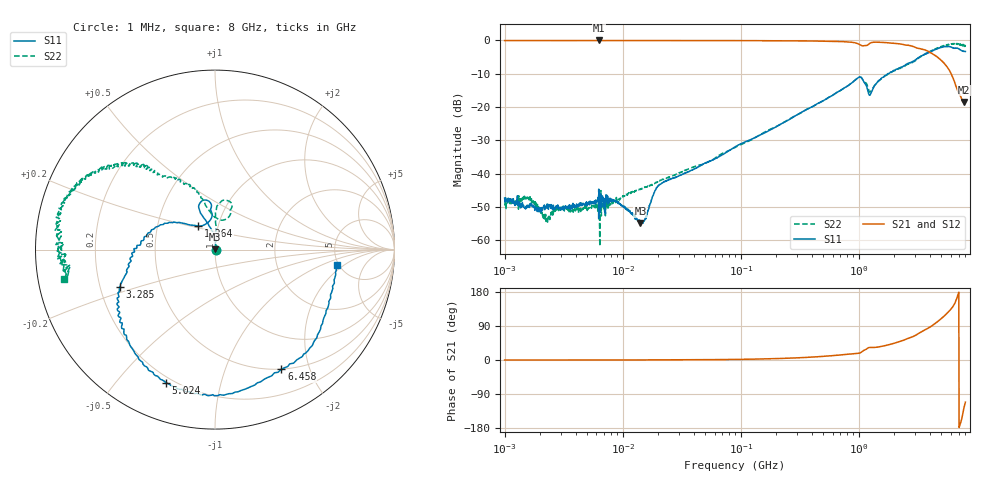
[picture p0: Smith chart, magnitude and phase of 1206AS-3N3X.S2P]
!s-Parameter Generated by FASTRON Sdn. Bhd.
!FASTRON P/N : 1206AS-3N3X
!Keysight Technologies: E5071C_MY46733604_B.14.02
!Date: Wed Nov 15 09:28:28 2023
!Version  :Rev00  Wed Nov 15 09:28:28 2023
!Data & Calibration Information:
!Freq  S11:SOLT2(ON)  S21:SOLT2(ON)  S12:SOLT2(ON)  S22:SOLT2(ON)
!PortZ  Port1:50+j0  Port2:50+j0
!When reading reference impedance value at option line is always used.
! Remarks : This data is being provided solely for informational purposes.
# Hz S dB R 50
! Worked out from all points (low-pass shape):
!   1601 points, 1 MHz to 8 GHz, reference 50 ohm
!   highest |S21| = 0.00 dB at 6.301 MHz (marker M1); lowest = -18.5 dB at 7.769 GHz (marker M2)
!   |S21| within 3 dB of the highest: start of sweep to 3.704 GHz
!   lowest |S11| = -54.9 dB at 14.15 MHz (marker M3), VSWR 1.00, Z = 50.1 + j0.125 ohm
!   |S11| at or under -10 dB: start of sweep to 1.756 GHz
!   |S22| runs from -61.8 to -0.9 dB; largest |S21 - S12| = 0.0043
!   S11 on the Smith chart (normalised r, x): 1 MHz: 1.01, -0.00; 1.264 GHz: 0.81, +0.22; 3.285 GHz: 0.28, -0.18; 5.024 GHz: 0.17, -0.68; 6.458 GHz: 0.50, -1.59; 8 GHz: 4.79, -1.55
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1000000  -47.36 -27.2  -0.02 -0.1  -0.04 -0.1  -49.23 -33.5
1568286  -50.06 -31.4  -0.02 -0.1  -0.03 -0.0  -47.04 -37.2
2286470  -49.17 8.8  -0.03 -0.0  -0.03 -0.0  -53.57 13.9
2905262  -50.51 4.0  -0.03 -0.0  -0.03 0.0  -50.89 1.5
4479405  -48.96 16.8  -0.03 0.0  -0.04 0.0  -50.94 21.6
6301378  -44.76 8.2  0.00 -0.1  -0.02 0.1  -49.76 -41.4
8860562  -48.44 31.0  -0.03 0.1  -0.03 0.1  -47.19 33.3
1.414737e7  -54.90 44.0  -0.03 0.2  -0.04 0.2  -44.58 35.3
1.552719e7  -53.42 55.5  -0.03 0.2  -0.04 0.2  -44.08 38.7
2.00676e7  -43.55 56.6  -0.03 0.3  -0.04 0.4  -42.34 57.9
8.994653e7  -31.93 81.2  -0.05 1.5  -0.06 1.5  -32.14 77.8
4.006501e8  -19.97 97.6  -0.15 7.7  -0.16 7.6  -19.96 87.2
1.007883e9  -11.03 104.9  -1.17 18.0  -1.18 18.0  -11.02 78.6
1.264475e9  -15.91 125.1  -0.70 33.1  -0.71 33.0  -15.26 85.1
1.7949e9  -9.92 153.8  -0.70 40.3  -0.71 40.1  -10.01 106.4
3.284549e9  -4.90 -158.4  -2.47 71.7  -2.49 71.7  -4.96 127.4
4.135839e9  -3.24 -136.3  -3.86 90.0  -3.85 90.0  -3.05 138.3
5.02444e9  -2.04 -110.2  -6.08 109.8  -6.06 109.7  -1.80 148.3
5.724236e9  -1.85 -88.1  -8.45 126.5  -8.43 126.2  -1.29 157.3
6.457806e9  -2.36 -60.9  -12.41 148.0  -12.39 147.6  -0.94 167.1
7.768671e9  -3.29 -14.2  -18.47 -127.6  -18.46 -128.1  -1.51 -176.0
8e9  -3.31 -7.2  -17.90 -111.1  -17.88 -111.6  -1.37 -169.1
